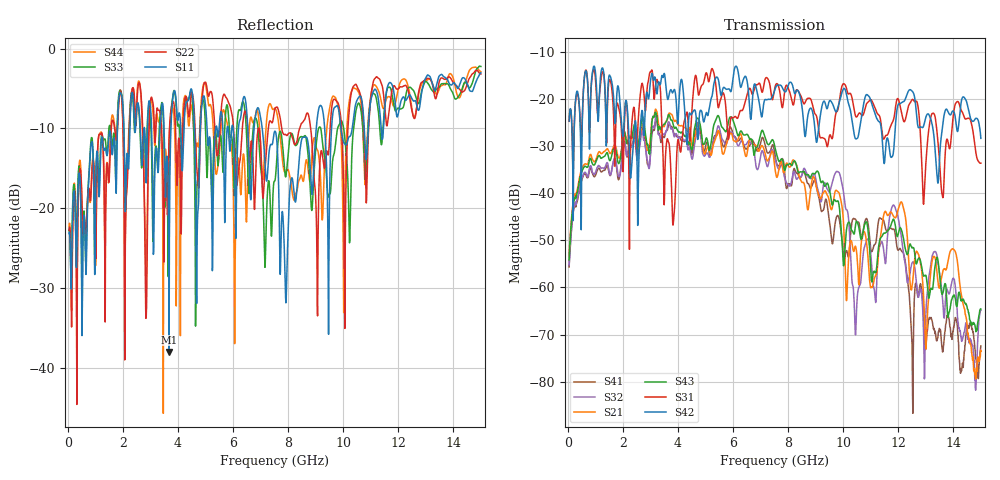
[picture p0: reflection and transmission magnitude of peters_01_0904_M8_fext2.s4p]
# MHZ S RI R 50.00
! FREQ  S11  S12  S13  S14
!  S21  S22  S23  S24
!  S31  S32  S33  S34
!  S41  S42  S43  S44
!  REAL  IMAG  REAL  IMAG  REAL  IMAG  REAL  IMAG
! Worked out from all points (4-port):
!   1496 points, 50 MHz to 15 GHz, reference 50 ohm
!   strongest paths, dB at 50 MHz, 3.79 GHz, 7.53 GHz, 11.27 GHz, 15 GHz:
!     S42: -24.7, -18.7, -17.9, -24.7, -28.4
!     S31: -24.8, -42.7, -17.4, -23.3, -33.7
!     S43: -54.2, -24.6, -30.4, -52.3, -64.6
!     S21: -53.3, -23.4, -35.0, -53.8, -73.6
!     S32: -55.2, -26.3, -32.9, -53.0, -64.8
!     S41: -55.7, -26.0, -32.1, -46.4, -72.4
!   lowest |S11| = -38.0 dB at 3.68 GHz (marker M1), VSWR 1.03, Z = 49.5 - j1.15 ohm
!   |S11| at or under -10 dB: start of sweep to 1.805 GHz; 7.061 GHz to 9.022 GHz (1.961 GHz wide, 24.4 % of centre); 9.916 GHz to 10.33 GHz (411.3 MHz wide, 4.06 % of centre)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
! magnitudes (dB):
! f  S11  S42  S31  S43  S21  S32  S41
! 50 MHz  -23.2  -24.7  -24.8  -54.2  -53.3  -55.2  -55.7
! 3.68 GHz  -38.0  -19.1  -29.5  -23.4  -23.1  -25.0  -25.5
! 7.92 GHz  -31.9  -18.4  -17.2  -34.4  -33.9  -37.5  -38.4
! 9.82 GHz  -7.4  -21.5  -22.0  -41.8  -39.8  -35.5  -44.8
! 10.45 GHz  -7.0  -28.5  -23.6  -46.8  -51.3  -70.1  -45.6
! 12.12 GHz  -6.4  -20.8  -23.0  -47.8  -41.9  -49.5  -52.3
! 15 GHz  -3.0  -28.4  -33.7  -64.6  -73.6  -64.8  -72.4
